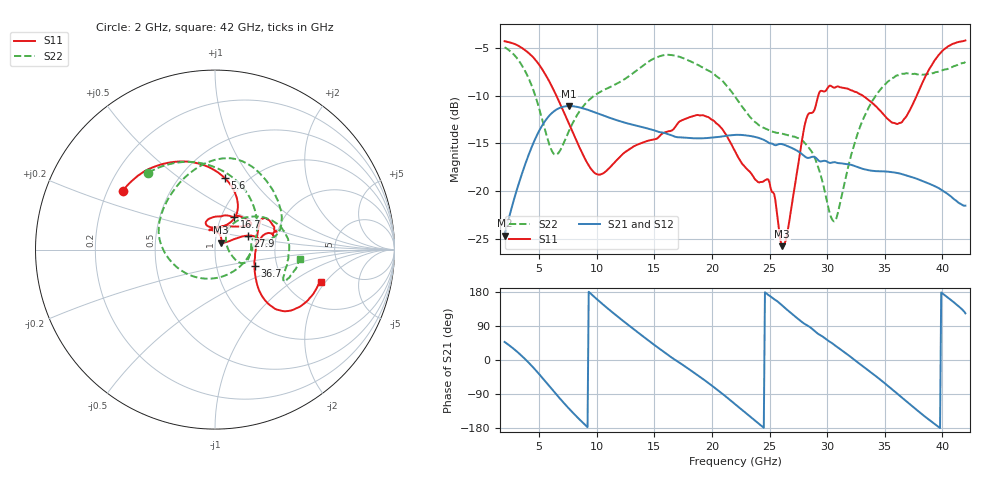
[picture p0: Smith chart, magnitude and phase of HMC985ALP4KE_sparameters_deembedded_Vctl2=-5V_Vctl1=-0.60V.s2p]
!s2p File: Measurements: S11, S21, S12, S22
# GHz S dB R 50.0
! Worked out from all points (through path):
!   401 points, 2 GHz to 42 GHz, reference 50 ohm
!   highest |S21| = -11.09 dB at 7.6 GHz (marker M1); lowest = -24.7 dB at 2 GHz (marker M2)
!   lowest |S11| = -25.8 dB at 26.1 GHz (marker M3), VSWR 1.11, Z = 53.4 + j4.1 ohm
!   |S11| at or under -10 dB: 6.492 GHz to 29.23 GHz (22.74 GHz wide, 127 % of centre); 33.09 GHz to 37.77 GHz (4.682 GHz wide, 13.2 % of centre)
!   |S22| runs from -23.2 to -4.9 dB; largest |S21 - S12| = 0.00029
!   S11 on the Smith chart (normalised r, x): 2 GHz: 0.26, +0.27; 5.6 GHz: 0.80, +0.76; 16.7 GHz: 1.15, +0.44; 27.9 GHz: 1.42, +0.23; 36.7 GHz: 1.53, -0.30; 42 GHz: 3.09, -1.77
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2  -4.30 147.3  -24.66 47.7  -24.66 47.7  -4.93 130.9
3.6  -5.09 120.7  -17.83 7.7  -17.84 7.7  -7.04 85.7
5.6  -7.91 82.2  -12.51 -58.6  -12.52 -58.6  -13.98 -5.0
6.5  -10.02 67.6  -11.45 -91.1  -11.46 -91.1  -16.16 -74.5
7.6  -12.96 58.5  -11.09 -128.7  -11.10 -128.7  -13.66 -140.0
8.7  -15.94 63.1  -11.29 -162.8  -11.30 -162.8  -11.30 -173.1
10.1  -18.25 88.1  -11.86 158.1  -11.87 158.1  -9.75 164.4
11.9  -16.54 109.5  -12.63 112.5  -12.64 112.5  -8.65 140.1
15.4  -14.31 77.4  -13.80 30.8  -13.81 30.9  -5.90 86.6
16.7  -13.46 59.6  -14.26 2.4  -14.26 2.4  -5.79 71.1
19.5  -12.18 35.1  -14.44 -56.4  -14.45 -56.4  -7.26 33.9
22  -15.80 52.6  -14.11 -116.3  -14.12 -116.3  -10.08 10.9
24.9  -18.80 100.6  -14.92 171.5  -14.92 171.6  -13.60 12.4
26.1  -25.75 47.9  -15.08 143.7  -15.09 143.8  -13.98 -0.8
27.9  -14.05 23.2  -16.21 98.3  -16.21 98.3  -14.75 -23.1
28.7  -11.79 11.5  -16.40 82.2  -16.41 82.3  -15.94 -27.6
30.7  -9.15 19.4  -16.97 38.0  -16.97 38.0  -23.10 24.4
32.9  -9.87 32.8  -17.59 -11.9  -17.60 -11.9  -13.12 50.2
35.4  -12.58 10.5  -17.97 -71.5  -17.98 -71.4  -8.42 21.1
36.7  -12.42 -22.4  -18.29 -104.5  -18.29 -104.5  -7.71 5.1
39.6  -5.89 -42.4  -19.63 -175.2  -19.63 -175.1  -7.51 -24.5
42  -4.22 -16.9  -21.51 123.2  -21.52 123.2  -6.46 -6.2
